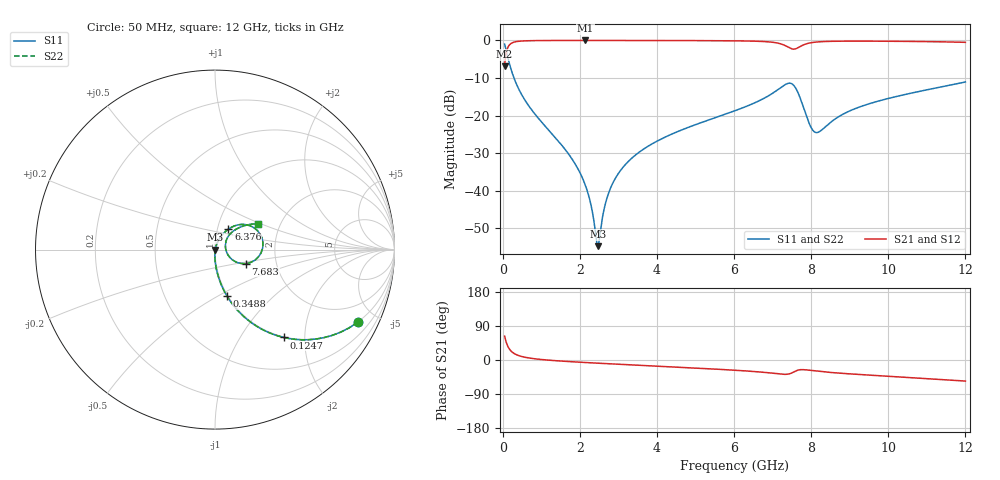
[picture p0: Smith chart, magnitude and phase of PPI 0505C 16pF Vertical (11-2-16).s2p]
# GHz S MA R 50
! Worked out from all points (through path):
!   1601 points, 50 MHz to 12 GHz, reference 50 ohm
!   highest |S21| = -0.02 dB at 2.141 GHz (marker M1); lowest = -6.9 dB at 50 MHz (marker M2)
!   group delay of S21, straight-line fit = 14.3 ps
!   lowest |S11| = -54.7 dB at 2.47 GHz (marker M3), VSWR 1.00, Z = 50.2 - j0.02 ohm
!   |S11| at or under -10 dB: 293.2 MHz to end of sweep
!   |S22| runs from -54.7 to -1.0 dB; largest |S21 - S12| = 0
!   S11 on the Smith chart (normalised r, x): 50 MHz: 0.99, -3.94; 124.7 MHz: 0.99, -1.58; 348.8 MHz: 0.99, -0.55; 6.376 GHz: 1.13, +0.26; 7.683 GHz: 1.39, -0.22; 12 GHz: 1.54, +0.48
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0.05  0.8927 -26.9  0.4505 63.0  0.4505 63.0  0.8927 -26.9
0.1246875  0.6212 -52.0  0.7833 38.0  0.7833 38.0  0.6212 -52.0
0.2143125  0.4171 -66.0  0.9083 23.9  0.9083 23.9  0.4171 -66.0
0.34875  0.2684 -75.5  0.9626 14.4  0.9626 14.4  0.2684 -75.5
0.8640937  0.1006 -86.6  0.9938 2.8  0.9938 2.8  0.1006 -86.6
2.044156  0.01576 -90.0  0.9981 -6.1  0.9981 -6.1  0.01576 -90.0
2.14125  0.01194 -88.4  0.9981 -6.6  0.9981 -6.6  0.01194 -88.4
2.275688  0.006985 -82.8  0.9981 -7.4  0.9981 -7.4  0.006985 -82.8
2.469875  0.001834 -6.2  0.998 -8.4  0.998 -8.4  0.001834 -6.2
2.693938  0.007675 65.9  0.9979 -9.6  0.9979 -9.6  0.007675 65.9
2.947875  0.01543 71.5  0.9977 -10.9  0.9977 -10.9  0.01543 71.5
3.381063  0.02807 72.4  0.9972 -13.1  0.9972 -13.1  0.02807 72.4
4.038312  0.04672 70.5  0.9961 -16.4  0.9961 -16.4  0.04672 70.5
6.025  0.1161 59.9  0.9866 -27.0  0.9866 -27.0  0.1161 59.9
6.376031  0.1362 56.7  0.9808 -29.3  0.9808 -29.3  0.1362 56.7
7.406719  0.2686 15.0  0.8118 -37.1  0.8118 -37.1  0.2686 15.0
7.683063  0.1884 -24.4  0.8112 -26.1  0.8112 -26.1  0.1884 -24.4
8.019156  0.06651 -12.6  0.9352 -27.9  0.9352 -27.9  0.06651 -12.6
8.190938  0.06027 15.5  0.9563 -29.9  0.9563 -29.9  0.06027 15.5
8.930344  0.1111 45.5  0.9773 -36.1  0.9773 -36.1  0.1111 45.5
10.01331  0.1696 43.4  0.9743 -43.0  0.9743 -43.0  0.1696 43.4
12  0.2798 30.9  0.9423 -55.6  0.9423 -55.6  0.2798 30.9
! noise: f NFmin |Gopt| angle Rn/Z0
0.05  0.0004195  0.8757  1.191  0.0007286
1.372  0.004379  0.6991  4.88  0.002842
2.701  0.007301  0.6549  9.179  0.004006
4.031  0.01023  0.6381  13.44  0.005262
5.36  0.01462  0.6609  17.72  0.008056
6.682  0.03274  0.7974  22.28  0.03222
8.012  0.07321  0.8871  26.84  0.1333
9.341  0.03413  0.7422  30.75  0.02473
10.67  0.03324  0.7076  34.55  0.02044
12  0.04524  0.7552  38.7  0.03332
